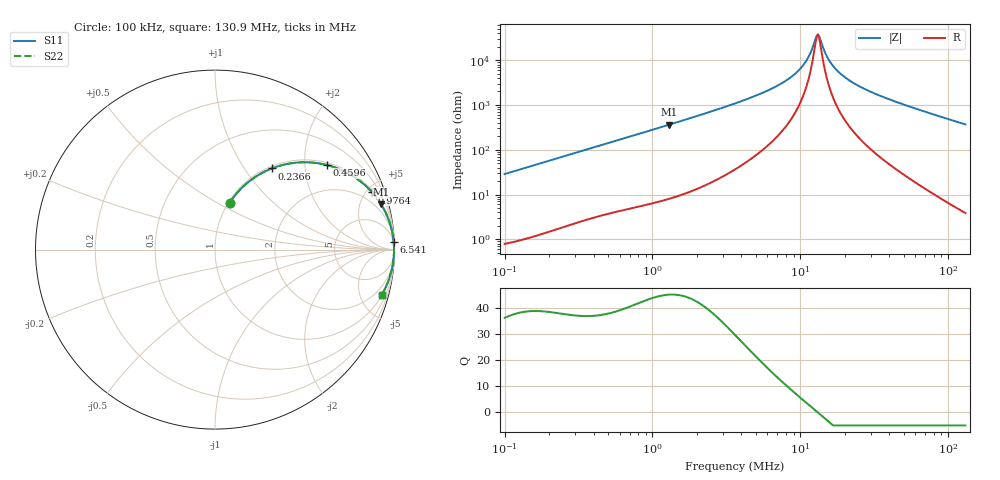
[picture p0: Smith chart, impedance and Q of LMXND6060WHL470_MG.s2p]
! LMXND6060WHL470_MG  S-PARAMETER MODEL  ( General Type )
! Model Generated by TAIYO YUDEN Corporation (http://www.ty-top.com)
! Version 1.0
! TAIYO YUDEN Control No. 191025NI43SB-FBB
! Copyright(c) 2019 TAIYO YUDEN CO.,LTD. All Rights Reserved.
! Product Description (link to TY-COMPAS)
! https://ds.yuden.co.jp/TYCOMPAS/or/detail?pn=LMXND6060WHL470MMG&u=M
! Products Name : Inductors
! Characteristics :
!  Inductance : 47 uH , SRF(min) : 8.0 MHz , DC Resistance(max) : 0.39 Ohm
!  Rated Current : Saturation :1000 mA , Temp Rise : 920 mA
!  Case Size : 6.0 x 6.0 / 0.236 x 0.236 [mm/inch] , Thickness : 2.8 / 0.11 [mm/inch]
!  (Conditions: Temperature = 25 degC , DC Bias Current/Voltage = 0A / 0V)
! External Node Assignments :
!  1  o---GGG---o  2
! GND o---------o GND
! Frequency Range : 0.1MHz  -  130.914307MHz  [ 402 STEP ]
# MHz S RI R 50
! Freq[MHz].  S11 Real  S11 Imag  S21 Real  S21 Imag  S12 Real  S12 Imag  S22 Real  S22 Imag
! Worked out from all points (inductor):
!   401 points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, 100 kHz to 130.9 MHz, reference 50 ohm
!   read as one part in series: L = 45.5 uH near 103.7 kHz
!   highest Q = 45.2 at 1.301 MHz (marker M1), where L = 44.5 uH
!   self-resonance near 12.93 MHz
!   S11 on the Smith chart (normalised r, x): 100 kHz: 1.02, +0.57; 236.6 kHz: 1.04, +1.34; 459.6 kHz: 1.07, +2.58; 976.4 kHz: 1.12, +5.45; 6.541 MHz: 4, +48; 130.9 MHz: 1.08, -7.35
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0.1  0.082 0.2609  0.918 -0.2609  0.918 -0.2609  0.082 0.2609
0.236613  0.3158 0.4519  0.6842 -0.4519  0.6842 -0.4519  0.3158 0.4519
0.332733  0.47 0.4858  0.53 -0.4858  0.53 -0.4858  0.47 0.4858
0.459579  0.622 0.4717  0.378 -0.4717  0.378 -0.4717  0.622 0.4717
0.976435  0.8757 0.3187  0.1243 -0.3187  0.1243 -0.3187  0.8757 0.3187
1.10711  0.9 0.2891  0.1 -0.2891  0.1 -0.2891  0.9 0.2891
1.301137  0.9249 0.2527  0.0751 -0.2527  0.0751 -0.2527  0.9249 0.2527
3.683715  0.9888 0.0893  0.0112 -0.0893  0.0112 -0.0893  0.9888 0.0893
6.541013  0.9955 0.0414  0.00449 -0.0414  0.00449 -0.0414  0.9955 0.0414
8.259373  0.9966 0.0264  0.00341 -0.0264  0.00341 -0.0264  0.9966 0.0264
9.706872  0.997 0.0169  0.00297 -0.0169  0.00297 -0.0169  0.997 0.0169
11.00592  0.9972 0.00978  0.00277 -0.00978  0.00277 -0.00978  0.9972 0.00978
12.03896  0.9973 0.00481  0.00269 -0.00481  0.00269 -0.00481  0.9973 0.00481
12.70476  0.9973 0.00186  0.00266 -0.00186  0.00266 -0.00186  0.9973 0.00186
13.16895  0.9973 -0.000113  0.00266 0.000113  0.00266 0.000113  0.9973 -0.000113
13.65011  0.9973 -0.00208  0.00266 0.00208  0.00266 0.00208  0.9973 -0.00208
14.66581  0.9973 -0.00603  0.00269 0.00603  0.00269 0.00603  0.9973 -0.00603
15.75709  0.9973 -0.01  0.00275 0.01  0.00275 0.01  0.9973 -0.01
18.85387  0.9969 -0.0202  0.00305 0.0202  0.00305 0.0202  0.9969 -0.0202
25.57835  0.9958 -0.0392  0.00418 0.0392  0.00418 0.0392  0.9958 -0.0392
40.05754  0.9918 -0.0742  0.0082 0.0742  0.0082 0.0742  0.9918 -0.0742
130.9143  0.9288 -0.2519  0.0712 0.2519  0.0712 0.2519  0.9288 -0.2519
